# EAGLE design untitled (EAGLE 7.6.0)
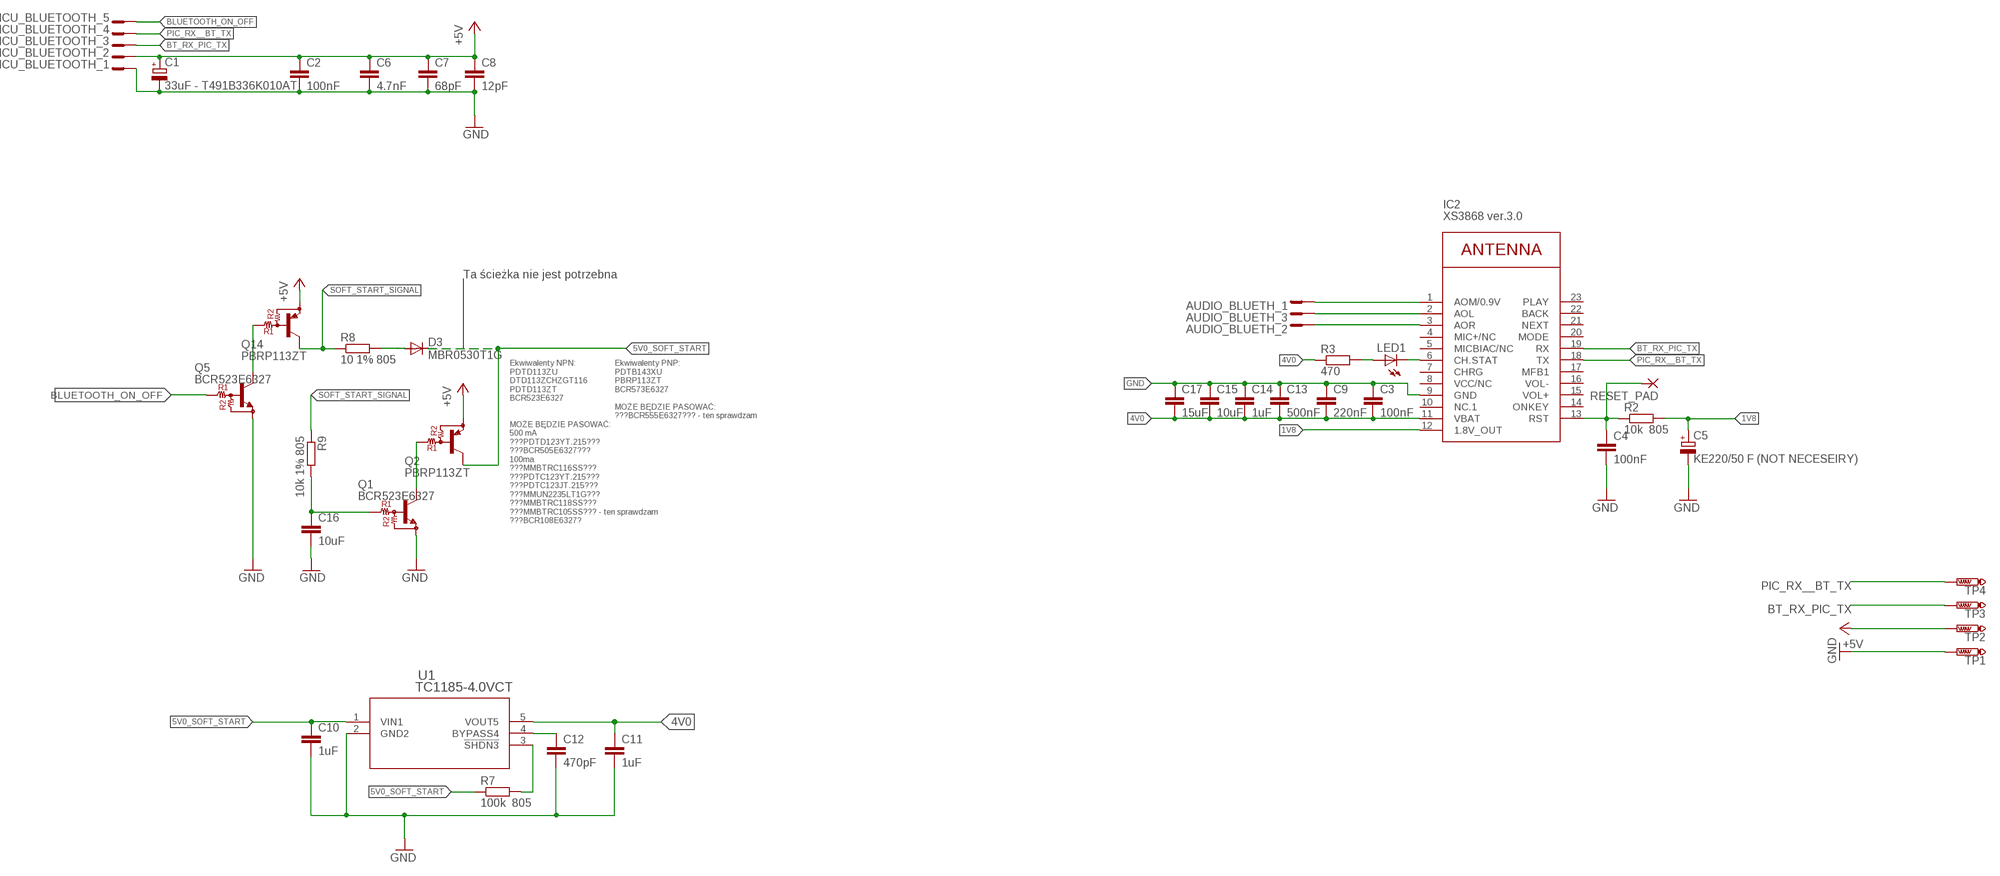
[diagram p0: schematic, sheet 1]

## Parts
AUDIO_BLUETH  JST_3_PIN_B3B-PH-KS  [B3B-PH-KS]
C1  33uF - T491B336K010AT  CPOL-EUSMCC  [SMC_C]
C2  100nF  C-EUC0805  [C0805]
C3  100nF  C-EUC0805  [C0805]
C4  100nF  C-EUC0805  [C0805]
C5  KE220/50 F (NOT NECESEIRY)  CPOL-EUG  [PANASONIC_G]
C6  4.7nF  C-EUC0805  [C0805]
C7  68pF  C-EUC0805  [C0805]
C8  12pF  C-EUC0805  [C0805]
C9  220nF  C-EUC0805  [C0805]
C10  1uF  C-EUC0805  [C0805]
C11  1uF  C-EUC0805  [C0805]
C12  470pF  C-EUC0805  [C0805]
C13  500nF  C-EUC0805  [C0805]
C14  1uF  C-EUC0805  [C0805]
C15  10uF  C-EUC0805  [C0805]
C16  10uF  C-EUC0805  [C0805]
C17  15uF  C-EUC0805  [C0805]
D3  MBR0530T1G  MBR0520LT  [SOD123]
IC2  XS3868 ver.3.0  WIRELESS-BLUETOOTH-XS3868  [WIRELESS-BLUETOOTH-XS3868]
LED1  LEDSML0805  [SML0805]
MCU_BLUETOOTH  JST_5_PIN_B5B-PH-KS  [B5B-PH-KS]
Q1  BCR523E6327  PDTD113ZU  [SOT-23]
Q2  PBRP113ZT  PDTB143XU  [SOT-23]
Q5  BCR523E6327  PDTD113ZU  [SOT-23]
Q14  PBRP113ZT  PDTB143XU  [SOT-23]
R2  10k 805  R-EU_M0805  [M0805]
R3  470  R-EU_M0805  [M0805]
R7  100k 805  R-EU_M0805  [M0805]
R8  10 1% 805  R-EU_M0805  [M0805]
R9  10k 1% 805  R-EU_M0805  [M0805]
RESET_PAD  SMD2  [SMD1,27-2,54]
TP1  PTR1B1,27  [B1,27]
TP2  PTR1B1,27  [B1,27]
TP3  PTR1B1,27  [B1,27]
TP4  PTR1B1,27  [B1,27]
U1  TC1185-4.0VCT  TC1185-X.XXCT713SOT-23-5_MC-M  [SOT-23-5_MC-M]

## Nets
1V8: C5.+ IC2.12(1.8V_OUT) R2.2
4V0: C3.2 C9.2 C11.1 C13.2 C14.2 C15.2 C17.2 IC2.11(VBAT) R3.1 U1.5(VOUT5)
5V0_SOFT_START: C10.1 D3.C Q2.3(C) R7.1 U1.1(VIN1)
+5V: C1.+ C2.1 C6.1 C7.1 C8.1 MCU_BLUETOOTH.P$2 Q2.2(E) Q14.2(E) TP2.TP
AUDIO_DIFF_COMMON: AUDIO_BLUETH.P$1 IC2.1(AOM/0.9V)
BLUETOOTH_ON_OFF: MCU_BLUETOOTH.P$5 Q5.1(B)
BT_LED: IC2.6(CH.STAT) LED1.C
BT_RX_PIC_TX: IC2.19(RX) MCU_BLUETOOTH.P$3 TP3.TP
BTOUT_LEFT: AUDIO_BLUETH.P$2 IC2.3(AOR)
BTOUT_RIGHT: AUDIO_BLUETH.P$3 IC2.2(AOL)
GND: C1.- C2.2 C3.1 C4.2 C5.- C6.2 C7.2 C8.2 C9.1 C10.2 C11.2 C12.2 C13.1 C14.1 C15.1 C16.2 C17.1 IC2.9(GND) MCU_BLUETOOTH.P$1 Q1.2(E) Q5.2(E) TP1.TP U1.2(GND2)
N$4: C12.1 U1.4(BYPASS4)
N$5: LED1.A R3.2
N$6: R7.2 U1.3(!SHDN3)
N$7: Q5.3(C) Q14.1(B)
N$8: C16.1 Q1.1(B) R9.2
N$9: Q1.3(C) Q2.1(B)
N$12: D3.A R8.2
PIC_RX__BT_TX: IC2.18(TX) MCU_BLUETOOTH.P$4 TP4.TP
RST: C4.1 IC2.13(RST) R2.1 RESET_PAD.1(P)
SOFT_START_SIGNAL: Q14.3(C) R8.1 R9.1
Unconnected: IC2.4(MIC+/NC) IC2.5(MICBIAC/NC) IC2.7(CHRG) IC2.8(VCC/NC) IC2.10(NC.1) IC2.14(ONKEY) IC2.15(VOL+) IC2.16(VOL-) IC2.17(MFB1) IC2.20(MODE) IC2.21(NEXT) IC2.22(BACK) IC2.23(PLAY)

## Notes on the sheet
- Ta ścieżka nie jest potrzebna
- Ekwiwalenty PNP:
  PDTB143XU
  PBRP113ZT
  BCR573E6327
  
  MOŻE BĘDZIE PASOWAĆ:
  ???BCR555E6327??? - ten sprawdzam
- Ekwiwalenty NPN:
  PDTD113ZU
  DTD113ZCHZGT116
  PDTD113ZT
  BCR523E6327
  
  
  MOŻE BĘDZIE PASOWAĆ:
  500 mA
  ???PDTD123YT.215???
  ???BCR505E6327???
  100ma
  ???MMBTRC116SS???
  ???PDTC123YT.215???
  ???PDTC123JT.215???
  ???MMUN2235LT1G???
  ???MMBTRC118SS???
  ???MMBTRC105SS??? - ten sprawdzam
  ???BCR108E6327?

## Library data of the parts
AUDIO_BLUETH = conn-JST:JST_3_PIN_
C1 = resistor:CPOL-EU: POLARIZED CAPACITOR, European symbol
C2-C4 C6-C15 C17 = resistor:C-EU: CAPACITOR, European symbol
C5 = rcl:CPOL-EU: POLARIZED CAPACITOR, European symbol
C16 = rcl:C-EU: CAPACITOR, European symbol
D3 = diode:MBR0520LT: SCHOTTKY BARRIER RECTIFIER
IC2 = diy-modules:WIRELESS-BLUETOOTH-XS3868: Bluetooth Stereo Audio Module based on OVC3860 chip More details available here: http://artofcircuits.com/product/bluetooth-2-0-edr-stereo-audio-ovc3860-module-model-xs-3868 Click here to find device on ebay.com
LED1 = led:LED: LED
MCU_BLUETOOTH = conn-JST:JST_5_PIN_
Q1 Q5 = pre-bias-transistor:PDTD: Pre biase NPN transistor NPN Resistor-Equipped Transistor (RET) family in a very small SOT323 (SC-70) Surface-Mounted Device (SMD) plastic package. VCC = 50V Ic (max) = 500 mA; R1: 1 kOhm; R2: 10 kOhm
Q2 Q14 = pre-bias-transistor:PDTB: PNP Resistor-Equipped Transistor (RET) family in a very small SOT323 (SC-70) Surface-Mounted Device (SMD) plastic package. VCC = -50 IC (max) = -500mA; R1: 4.7 kOhm; R2: 10 kOhm
R2 R3 R7-R9 = rcl:R-EU_: RESISTOR, European symbol
RESET_PAD = wirepad:SMD2: SMD PAD
TP1-TP4 = testpad:PTR1: TEST PIN
U1 = TC1185:TC1185-X.XXCT713; MANUFACTURER_PART_NUMBER: TC1185X.XXCT713; VENDOR: Microchip

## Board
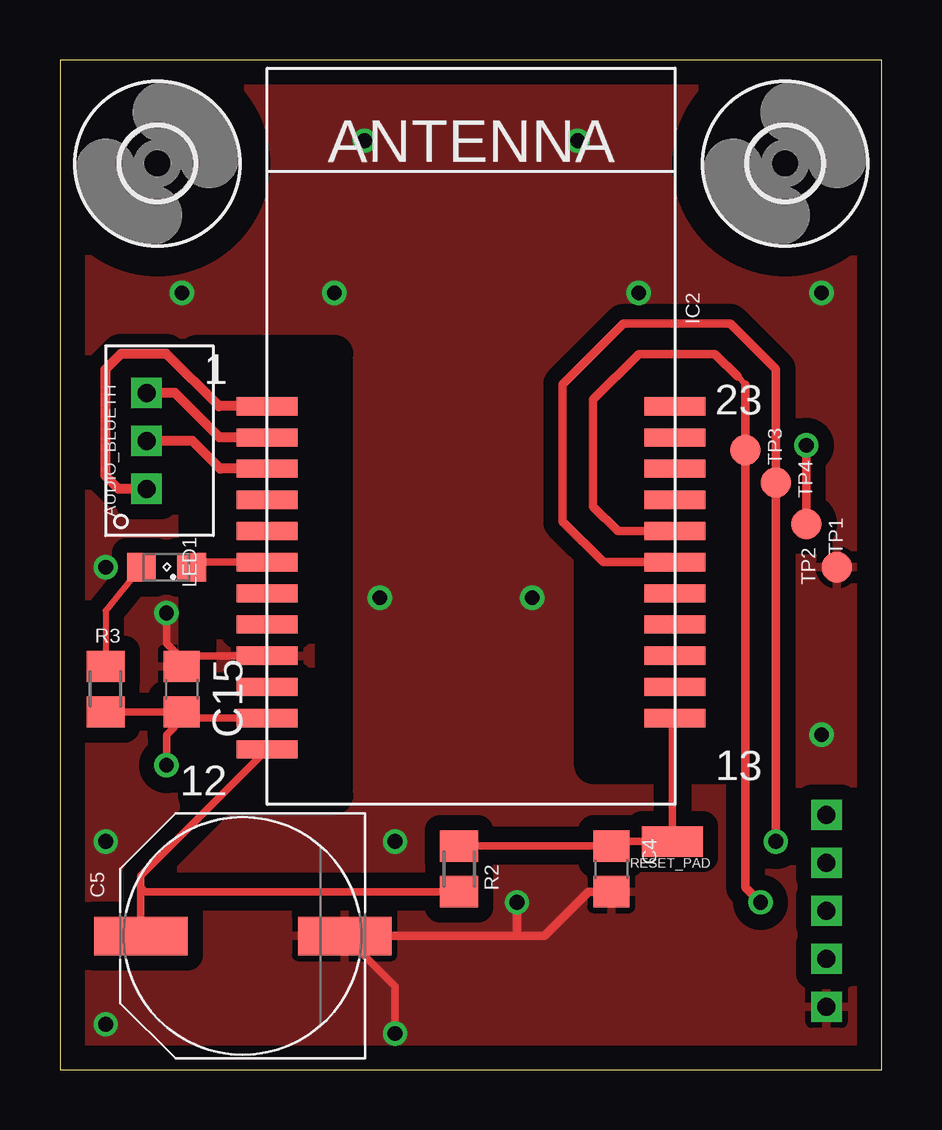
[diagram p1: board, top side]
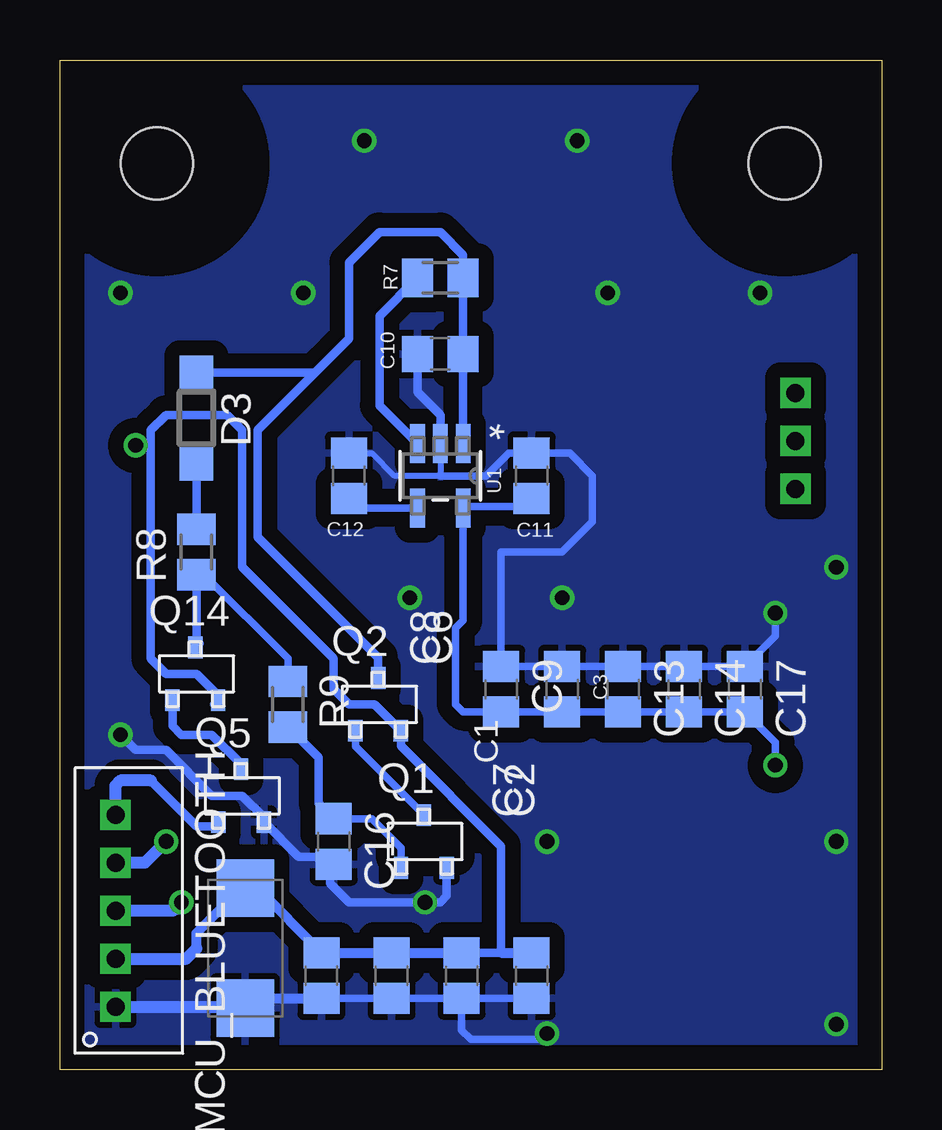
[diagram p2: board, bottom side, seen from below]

Size 34.27 x 42.1 mm. Coordinates in mm from the lower left corner, seen from the top.
Outline: 0,0 34.27,0 34.27,42.1 0,42.1 0,0
Copper layers (1*16): Top 0.035mm / dielectric 1.5mm / Bottom 0.035mm
Design rules "default": minimum track width 10mil, minimum drill 24mil, track to track 8mil, track to pad 8mil, pad to pad 8mil, via to via 8mil, smd to smd 8mil, copper to edge 40mil, drill to drill 8mil, minimum pad ring 10mil, minimum via ring 8mil, stop-mask expansion 4mil, vias tented up to drill 0mil, thermal gap 10mil
tRestrict: 8 lines
bRestrict: area 17.8,8.9 to 20.3,8.9

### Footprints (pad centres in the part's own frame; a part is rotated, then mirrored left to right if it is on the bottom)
B3B-PH-KS = drill 0.75 pad 1.2 square: P$1 -2,1.7; P$2 -4,1.7; P$3 -6,1.7
SMC_C = smd 2.4 x 2.4: + -2.5,0; - 2.5,0
C0805 = smd 1.3 x 1.5: 1 -0.95,0; 2 0.95,0
PANASONIC_G = smd 3.9 x 1.6: + 4.25,0; - -4.25,0
SOD123 = smd 1.4 x 1.4: A 1.9,0; C -1.9,0
WIRELESS-BLUETOOTH-XS3868 = smd 2.54 x 0.762: 1 -8.5,0.995; 2 -8.5,-0.305; 3 -8.5,-1.605; 4 -8.5,-2.905; 5 -8.5,-4.205; 6 -8.5,-5.505; 7 -8.5,-6.805; 8 -8.5,-8.105; 9 -8.5,-9.405; 10 -8.5,-10.705; 11 -8.5,-12.005; 12 -8.5,-13.305; 13 8.5,-12.005; 14 8.5,-10.705; 15 8.5,-9.405; 16 8.5,-8.105; 17 8.5,-6.805; 18 8.5,-5.505; 19 8.5,-4.205; 20 8.5,-2.905; 21 8.5,-1.605; 22 8.5,-0.305; 23 8.5,0.995
SML0805 = smd 1.2 x 1.2: A 1.05,0; C -1.05,0
B5B-PH-KS = drill 0.75 pad 1.2 square: P$1 -2,1.7; P$2 -4,1.7; P$3 -6,1.7; P$4 -8,1.7; P$5 -10,1.7
SOT-23 = smd 0.6 x 0.9: 1 -1,-1.1; 2 0.9,-1.1; 3 -0.05,1.1
M0805 = smd 1.3 x 1.6: 1 -0.95,0; 2 0.95,0
SMD1,27-2,54 = smd 1.27 x 2.54: 1 0,0
B1,27 = smd 1.27 x 1.27: TP 0,0
SOT-23-5_MC-M = smd 1.626 x 0.61: 1 -1.346,0.95; 2 -1.346,0; 3 -1.346,-0.95; 4 1.346,-0.95; 5 1.346,0.95
3,0 = hole 3: 0,0

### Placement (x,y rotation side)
AUDIO_BLUETH  1.9,22.23 270 top
C1  26.54,5.08 270 bottom
C2  23.37,3.94 270 bottom
C3  13.33,15.88 270 bottom
C4  22.99,8.38 270 top
C5  7.62,5.59 180 top
C6  20.45,3.94 270 bottom
C7  17.53,3.94 270 bottom
C8  14.6,3.94 270 bottom
C9  15.87,15.88 270 bottom
C10  18.41,29.84 180 bottom
C11  14.6,24.77 90 bottom
C12  22.23,24.77 90 bottom
C13  10.79,15.88 270 bottom
C14  8.26,15.88 270 bottom
C15  5.08,15.88 270 top
C16  22.86,9.52 270 bottom
C17  5.71,15.88 270 bottom
D3  28.57,27.18 270 bottom
IC2  17.14,26.67 0 top
LED1  4.44,20.96 180 top
MCU_BLUETOOTH  33.65,0.63 270 bottom
Q1  19.05,9.52 0 bottom
Q2  20.95,15.24 0 bottom
Q5  26.67,11.43 0 bottom
Q14  28.57,16.51 0 bottom
R2  16.64,8.38 270 top
R3  1.9,15.88 90 top
R7  18.41,33.02 180 bottom
R8  28.57,21.59 90 bottom
R9  24.77,15.24 270 bottom
RESET_PAD  25.53,9.52 270 top
TP1  32.38,20.96 0 top
TP2  31.11,22.77 0 top
TP3  28.57,25.85 0 top
TP4  29.84,24.48 0 top
U1  18.41,24.77 270 bottom
U$2  [3,0]  4.06,37.78 0 top
U$3  [3,0]  30.23,37.78 0 top

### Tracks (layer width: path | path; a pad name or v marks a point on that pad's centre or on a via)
1V8
  Top 0.305: IC2.12 3.37,8.09 3.37,7.62 | 3.37,7.62 C5.+ | R2.2 3.56,7.43 3.37,7.62
4V0  (via drill 0.61)
  Top 0.305: C15.2 R3.1 | IC2.11 5.34,14.66 C15.2 | C15.2 5.08,14.61 4.44,13.97 v4.44,12.7
  Bottom 0.305: C17.2 5.4,14.93 | C17.2 C14.2 C13.2 C3.2 C9.2 17.46,14.93 17.78,15.24 17.78,18.41 17.46,18.73 U1.5 17.39,23.5 14.6,23.5 C11.1 | v4.44,12.7 4.44,13.66 C17.2
5V0_SOFT_START
  Bottom 0.356: 28.07,28.57 D3.C 23.63,29.08 | Q2.3 21.01,17.2 26.03,22.23 26.03,26.67 23.63,29.08 | U1.1 C10.1 R7.1 17.46,33.98 18.41,34.93 20.95,34.93 22.23,33.66 22.23,30.48 23.49,29.21 23.63,29.08
+5V  (via drill 0.61)
  Top 0.356: TP2.TP v31.11,26.04
  Bottom 0.356: 15.02,5.3 C8.1 | 27.84,15.24 Q14.2 27.67,15.61 28.57,16.51 29.84,16.51 30.48,17.14 30.48,26.04 | v31.11,26.04 30.48,26.04 | C7.1 15.87,4.89 15.87,9.32 20.05,13.51 Q2.2 21.16,15.24 22.23,15.24 22.86,15.88 22.86,17.14 26.67,20.96 26.67,26.67 27.3,27.3 29.84,27.3 30.48,26.67 30.48,26.04
  Bottom 0.406: C7.1 C6.1 C2.1 | C2.1 23.85,4.89 | C2.1 26.06,7.58 C1.+ 26.54,7.09 27.2,7.09 28.57,5.72 28.57,5.06 | 15.87,4.89 C8.1
  Bottom 0.508: MCU_BLUETOOTH.P$2 29,4.63 28.57,5.06
AUDIO_DIFF_COMMON
  Top 0.406: IC2.1 6.62,27.66 4.44,29.84 2.54,29.84 1.9,29.21 1.9,24.77 2.44,24.23 AUDIO_BLUETH.P$1
BLUETOOTH_ON_OFF
  Bottom 0.356: Q5.1 27.84,10.16 28.57,10.16 30.48,12.07
  Bottom 0.508: 30.48,12.07 31.75,12.07 31.95,11.86 MCU_BLUETOOTH.P$5
BT_LED
  Top 0.305: LED1.C 5.71,21.16 IC2.6
BT_RX_PIC_TX  (via drill 0.61)
  Top 0.254: TP3.TP 28.57,28.57 28.26,28.89
  Top 0.356: IC2.19 23.26,22.46 22.23,23.5 22.23,27.94 24.13,29.84 27.3,29.84 28.26,28.89 | 28.57,28.57 28.57,7.62 v29.21,6.99
  Bottom 0.508: v29.21,6.99 29.56,6.64 MCU_BLUETOOTH.P$3
BTOUT_LEFT
  Top 0.406: IC2.3 6.68,25.07 5.52,26.23 AUDIO_BLUETH.P$2
BTOUT_RIGHT
  Top 0.406: IC2.2 6.65,26.37 4.79,28.23 AUDIO_BLUETH.P$3
GND  (via drill 0.61)
  Top 0.305: IC2.9 5.52,17.27 C15.1 5.08,17.14 4.44,17.78 v4.44,19.05 | 12.06,5.39 C5.- 13.97,3.49 v13.97,1.52
  Top 0.356: C4.2 22.04,7.43 20.19,5.59 19.05,5.59 | 19.05,5.59 C5.- | v19.05,6.99 19.05,5.59
  Bottom 0.254: U1.2 18.41,24.77 20.32,24.77 21.27,25.71 C12.2
  Bottom 0.305: C2.2 C6.2 C7.2 | C17.1 C14.1 C13.1 C3.1 C9.1 15.87,21.59 13.33,21.59 12.06,22.86 12.06,24.77 13.01,25.71 C11.2 15.56,25.71 16.51,24.77 18.41,24.77 | C17.1 5.39,17.14 | v4.44,19.05 4.44,18.1 C17.1 | C7.2 C8.2 | C7.2 17.53,1.65 17.14,1.27 14.22,1.27 v13.97,1.52
  Bottom 0.356: 23.01,8.43 C16.2 | 23.01,8.43 23.01,7.77 22.23,6.99 v19.05,6.99 18.41,6.99 18.15,7.25 Q1.2 | U1.2 18.41,27.3 19.37,28.26 C10.2 | 23.01,8.43 23.48,8.89 24.33,8.89 Q5.2 25.77,10.53 26.67,11.43 27.94,11.43 29.84,13.34 31.11,13.34 v31.75,13.97
  Bottom 0.406: C2.2 25.53,2.99 C1.- 26.79,2.63
  Bottom 0.508: MCU_BLUETOOTH.P$1 26.79,2.63
  other vias: 5.08,32.38 31.75,32.38 1.9,1.91 1.9,9.52 13.97,9.52 11.43,32.38 24.13,32.38 13.33,19.69 19.69,19.69 12.7,38.73 21.59,38.73 1.9,20.96
  pour Bottom (isolate 0.635): -1.91,24.13 -1.91,43.18 36.2,43.18 36.2,-1.27 -0.64,-1.27 -1.91,-1.27
  pour Top (isolate 0.635): -1.91,22.86 -1.91,43.18 36.2,43.18 36.2,-1.27 -1.91,-1.27
N$4
  Bottom 0.305: U1.4 21.83,23.42 C12.1
N$5
  Top 0.254: LED1.A 1.9,19.14 R3.2
N$6
  Bottom 0.356: R7.2 20.95,31.43 20.95,27.7 U1.3
N$7
  Bottom 0.356: Q5.3 26.72,12.75 27.94,13.97 29.21,13.97 29.57,14.34 Q14.1
N$8
  Bottom 0.305: Q1.1 20.05,9.25 21.27,10.48 C16.1
  Bottom 0.356: C16.1 23.49,11.11 23.49,13.02 R9.2
N$9
  Bottom 0.305: Q1.3 21.95,13.48 Q2.1
N$12
  Bottom 0.356: D3.A R8.2
PIC_RX__BT_TX  (via drill 0.61)
  Top 0.254: TP4.TP 29.84,29.21
  Top 0.356: IC2.18 22.65,21.16 20.95,22.86 20.95,28.57 23.49,31.12 27.94,31.12 29.84,29.21 v29.84,9.52
  Bottom 0.508: v29.84,9.52 30.73,8.64 MCU_BLUETOOTH.P$4
RST
  Top 0.305: IC2.13 25.53,14.66 RESET_PAD.1 23.18,9.52 C4.1 R2.1
SOFT_START_SIGNAL
  Bottom 0.305: R9.1 24.77,17.14 28.26,20.64 R8.1
  Bottom 0.356: R8.1 28.57,17.66 Q14.3 28.45,17.78 | 25.09,16.51 R9.1

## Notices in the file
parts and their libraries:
diy-modules: Released under the Creative Commons Attribution 4.0 International License: http://creativecommons.org/licenses/by/4.0
